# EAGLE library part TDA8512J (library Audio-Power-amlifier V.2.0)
The TDA8512J is an integrated class-B output amplifier in a 17-lead Single-In-Line (SIL) power package. It contains 4 ´ 13 WSingle Ended (SE) amplifiers of which two can be used to configure a 26 W BTL amplifier.
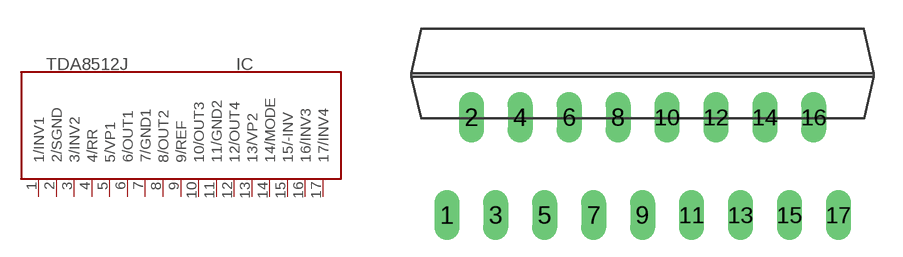
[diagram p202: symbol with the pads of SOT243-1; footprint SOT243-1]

Designator prefix IC

## TDA8512J  [SOT243-1]
1  1/INV1  in
2  2/SGND  pwr
3  3/INV2  in
4  4/RR
5  5/VP1  pwr
6  6/OUT1  out
7  7/GND1  pwr
8  8/OUT2  out
9  9/REF  in
10  10/OUT3  out
11  11/GND2  pwr
12  12/OUT4  out
13  13/VP2  pwr
14  14/MODE  in
15  15/-INV  in
16  16/INV3  in
17  17/INV4  in

## Footprint SOT243-1 (pad centres in mm)
DBS17P: plastic DIL-bent-SIL power package; 17 leads (lead length 7.7 mm)
drill 0.8 long: 1 -10.16,-5.08; 2 -8.89,0; 3 -7.62,-5.08; 4 -6.35,0; 5 -5.08,-5.08; 6 -3.81,0; 7 -2.54,-5.08; 8 -1.27,0; 9 0,-5.08; 10 1.27,0; 11 2.54,-5.08; 12 3.81,0; 13 5.08,-5.08; 14 6.35,0; 15 7.62,-5.08; 16 8.89,0; 17 10.17,-5.08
